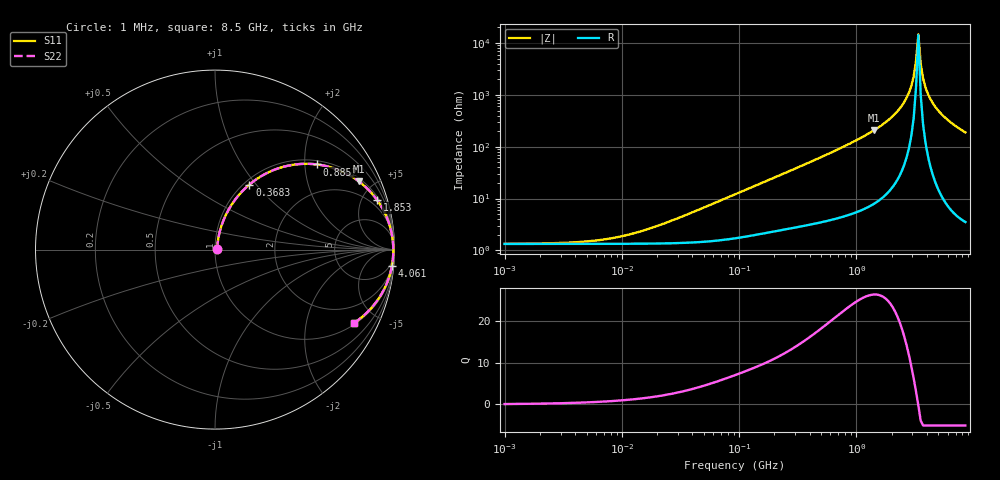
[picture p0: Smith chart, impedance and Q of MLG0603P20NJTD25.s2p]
! S-Parameter Data Generated by TDK Corporation
! Copyright(C) 2025 TDK Corporation.
! All Rights Reserved.
! TDK P/N: MLG0603P20NJTD25 (SMD / SMT Inductor (Coil))
! Property: L=20nH at 500MHz
! Size(LxWxT): 0.6x0.3x0.3mm
! Model Type: s2p (Touchstone File Format Version 1.0)
! Frequency: DC=Yes Start=1MHz Stop=8500MHz 198points Log-sweep
! Model Generated on Feb. 6, 2025
! Terms and conditions regarding TDK Simulation Models:
! 1)This simulation model is being provided solely for informational
!  purposes. Please refer to the specifications of the products in
!  terms of detailed characteristics of such products.
! 2)In no event shall TDK Corporation of any of its subsidiaries be
!  liable for any loss or damage arising, directly or indirectly,
!  from any information contained in this simulation model, including,
!  but not limited to loss or damages arising from any inaccuracies,
!  omissions or errors in connection with such information.
! 3)Any and all copyrights on this simulation model are owned by
!  TDK Corporation.  Duplication or redistribution of this simulation
!  model without prior written permission from TDK Corporation
!  is prohibited.
! 4)This simulation model is subject to any modification or change
!  without any prior notice.
! 5)Neither TDK Corporation nor any of its subsidiaries shall make any
!  warranty, express or implied, including but not limited to the
!  correctness, implied warranties of merchantability and fitness for
!  a particular purpose with respect to this simulation models.
! 6)The use of this simulation model shall be deemed to have consented
!  to the terms and conditions hereof.
! Port Assignments:
!  1 ---@@@--- 2
! Applicable Conditions:
!  Temperature = 25 degC
!  DC Bias Current = 0 A
!  Small Signal Operation
# Hz S MA R 50
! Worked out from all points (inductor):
!   197 points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, 1 MHz to 8.5 GHz, reference 50 ohm
!   read as one part in series: L = 20.8 nH near 31.89 MHz
!   highest Q = 26.2 at 1.405 GHz (marker M1), where L = 23.3 nH
!   self-resonance near 3.224 GHz
!   S11 on the Smith chart (normalised r, x): 1 MHz: 1.03, +0.00; 368.3 MHz: 1.06, +0.92; 885.2 MHz: 1.10, +2.31; 1.853 GHz: 1.26, +6.41; 4.061 GHz: 2, -21; 8.5 GHz: 1.07, -3.78
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1000000  0.01319 5.6  0.9869 -0.1  0.9869 -0.1  0.01319 5.6
4587603  0.01442 24.0  0.9868 -0.3  0.9868 -0.3  0.01442 24.0
1.005548e7  0.01853 43.9  0.9867 -0.7  0.9867 -0.7  0.01853 43.9
2.10461e7  0.03033 62.3  0.9863 -1.6  0.9863 -1.6  0.03033 62.3
9.219544e7  0.1175 75.2  0.9766 -6.7  0.9766 -6.7  0.1175 75.2
3.682571e8  0.4095 62.2  0.8861 -24.1  0.8861 -24.1  0.4095 62.2
4.229561e8  0.4577 59.4  0.8619 -27.2  0.8619 -27.2  0.4577 59.4
8.852465e8  0.7414 39.8  0.6403 -47.8  0.6403 -47.8  0.7414 39.8
1.404574e9  0.8862 25.5  0.4307 -62.3  0.4307 -62.3  0.8862 25.5
1.852819e9  0.9439 17.1  0.2943 -70.6  0.2943 -70.6  0.9439 17.1
1.940355e9  0.9513 15.7  0.2714 -71.9  0.2714 -71.9  0.9513 15.7
2.559585e9  0.9826 7.7  0.1346 -78.7  0.1346 -78.7  0.9826 7.7
2.939772e9  0.9905 3.8  0.06662 -79.9  0.06662 -79.9  0.9905 3.8
3.07866e9  0.9921 2.5  0.04411 -78.4  0.04411 -78.4  0.9921 2.5
3.224109e9  0.993 1.2  0.02194 -70.9  0.02194 -70.9  0.993 1.2
3.37643e9  0.9935 -0.1  0.006773 15.3  0.006773 15.3  0.9935 -0.1
3.535948e9  0.9934 -1.4  0.02532 74.1  0.02532 74.1  0.9934 -1.4
3.703002e9  0.9927 -2.7  0.04765 79.8  0.04765 79.8  0.9927 -2.7
4.061159e9  0.9897 -5.3  0.09304 81.0  0.09304 81.0  0.9897 -5.3
4.664383e9  0.981 -9.3  0.1618 78.6  0.1618 78.6  0.981 -9.3
5.357206e9  0.9669 -13.4  0.2312 75.2  0.2312 75.2  0.9669 -13.4
8.5e9  0.8773 -27.6  0.4639 61.3  0.4639 61.3  0.8773 -27.6
